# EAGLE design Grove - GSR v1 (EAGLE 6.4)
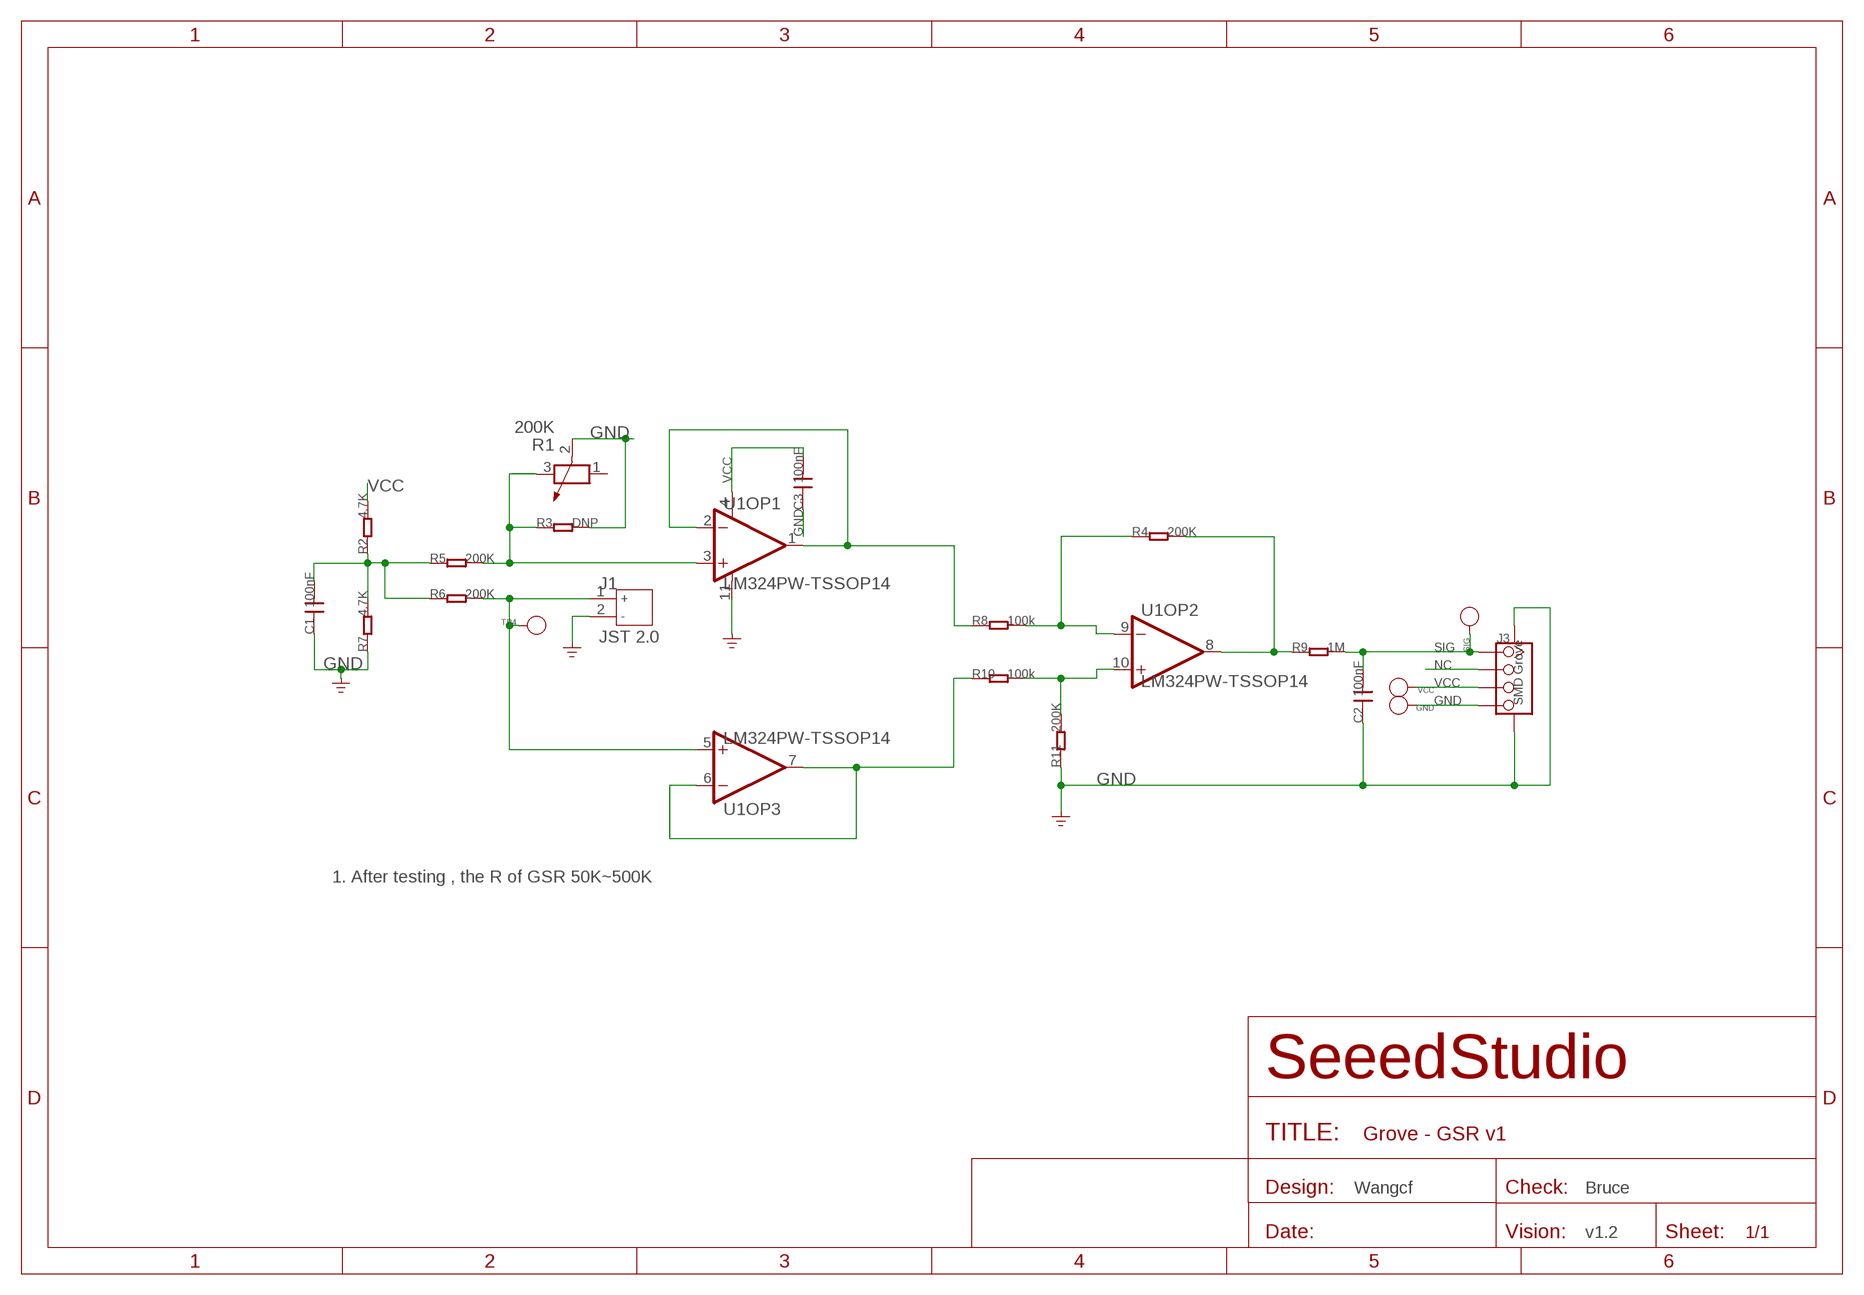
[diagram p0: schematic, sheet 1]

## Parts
C1  100nF  C-0603  [0603]
C2  100nF  C-0603  [0603]
C3  100nF  C-0603  [0603]
GND  PAD-TEST-POINT'4545'  [TP_4545]
J1  JST 2.0  JACK-JST-2P-PW'2.0'  [JST-2.0]
J3  SMD Grove  TWIG-4P-2.0-SMD-FEMALE-REINFORCE'DD'  [4P-SMD-2.0]
R1  200K  R-POTENTIOMETER-SMD  [3P-SMD-RECT-3.3X3.6]
R2  4.7K  R-0603  [0603]
R3  DNP  R-0603  [0603]
R4  200K  R-0603  [0603]
R5  200K  R-0603  [0603]
R6  200K  R-0603  [0603]
R7  4.7K  R-0603  [0603]
R8  100k  R-0603  [0603]
R9  1M  R-0603  [0603]
R10  100k  R-0603  [0603]
R11  200K  R-0603  [0603]
SIG  PAD-TEST-POINT'4545'  [TP_4545]
TP4  PAD-TEST-POINT'4545'  [TP_4545]
U1  LM324PW-TSSOP14  LMV324-TSSOP14  [TSSOP14]
VCC  PAD-TEST-POINT'4545'  [TP_4545]

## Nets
GND: C1.1 C2.1 C3.1 GND.T J1.2 J3.4 J3.SS1 J3.SS2 R1.2 R3.2 R7.1 R11.1 U1.11(OP1:V-)
IN: J1.1 R6.2 TP4.T U1.5(OP3:IN+)
N$1: R8.1 U1.1(OP1:OUT) U1.2(OP1:IN-)
N$2: R10.1 U1.6(OP3:IN-) U1.7(OP3:OUT)
N$3: R4.1 R8.2 U1.9(OP2:IN-)
N$4: R4.2 R9.1 U1.8(OP2:OUT)
N$5: R10.2 R11.2 U1.10(OP2:IN+)
N$6: C1.2 R2.1 R5.1 R6.1 R7.2
N$8: R1.3 R3.1 R5.2 U1.3(OP1:IN+)
NC: J3.2
SIG: C2.2 J3.1 R9.2 SIG.T
VCC: C3.2 J3.3 R2.2 U1.4(OP1:V+) VCC.T
Unconnected: R1.1 U1.12(OP4:IN+) U1.13(OP4:IN-) U1.14(OP4:OUT)

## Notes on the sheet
- 1. After testing , the R of GSR 50K~500K
- Wangcf | Bruce
- v1.2

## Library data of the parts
C1-C3 = Discreter:C*: Ceramic Capacitors
GND SIG TP4 VCC = Discrete:PAD-TEST-POINT; PARTNO: DNP
J1 = Connector:JACK-JST-2P-PW
J3 = Connector:TWIG-4P-2.0-SMD-FEMALE-REINFORCE
R1 = Discreter:R-POTENTIOMETER*: Potentiometer
R2-R11 = Discreter:R*
U1 = IC:LMV324: General purpose LOW Voltage, Rail-to-Rail Output Amplifiers http://www.fairchildsemi.com/ds/LM/LMV358.pdf

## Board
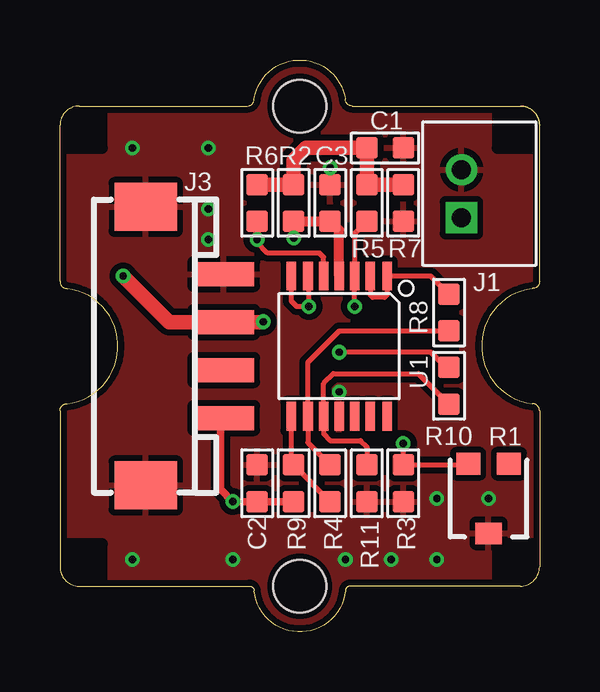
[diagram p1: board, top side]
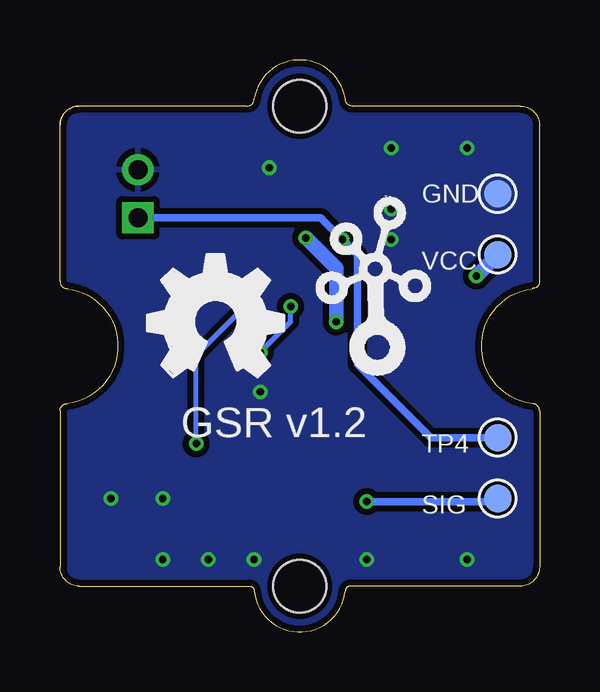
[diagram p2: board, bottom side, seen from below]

Size 20 x 23.83 mm. Coordinates in mm from the lower left corner, seen from the top.
Copper layers (1*16): Top 0.035mm / dielectric 1.5mm / Bottom 0.035mm
Design rules "SeeedStudio_rule_no_angle_090911 *": minimum track width 6mil, minimum drill 12mil, track to track 6mil, track to pad 6mil, pad to pad 6mil, via to via 6mil, smd to smd 0mil, copper to edge 10mil, drill to drill 10mil, minimum pad ring 10mil, minimum via ring 6mil, stop-mask expansion 2mil, vias tented up to drill 100mil, thermal gap 10mil

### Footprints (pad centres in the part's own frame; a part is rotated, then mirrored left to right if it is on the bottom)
0603 = smd 0.889 x 0.889: 1 -0.762,0; 2 0.762,0
TP_4545 = smd 1.143 x 1.143: T 0,0
JST-2.0 = drill 0.8 pad 1.3 square: 1 -1,0.75 | drill 0.8 pad 1.3: 2 1,0.75
4P-SMD-2.0 = smd 1 x 2.54: 1 -3,0; 2 -1,0; 3 1,0; 4 3,0 | smd 2 x 2.6: SS1 -5.8,3.25; SS2 5.8,3.25
3P-SMD-RECT-3.3X3.6 = smd 1 x 0.9: 1 -0.85,-1.45; 3 0.85,-1.45 | smd 1.1 x 0.9: 2 0,1.45
TSSOP14 = smd 0.4 x 1.2: 1 -2,-2.925; 2 -1.3,-2.925; 3 -0.65,-2.925; 4 0,-2.925; 5 0.65,-2.925; 6 1.3,-2.925; 7 2,-2.925; 8 2,2.925; 9 1.3,2.925; 10 0.65,2.925; 11 0,2.925; 12 -0.65,2.925; 13 -1.3,2.925; 14 -2,2.925
1U-DIM-W/-DRILL = hole 2.2: 0,-10; 0,10

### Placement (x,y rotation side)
C1  13.56,20.16 180 top
C2  8.22,6.19 270 top
C3  11.27,17.88 270 top
GND  1.74,18.26 0 bottom
J1  17.49,18.26 90 top
J3  6.83,11.91 90 top
R1  17.87,5.56 180 top
R2  9.75,17.88 270 top
R3  14.32,6.19 270 top
R4  11.27,6.19 270 top
R5  12.79,17.88 270 top
R6  8.22,17.88 270 top
R7  14.32,17.88 90 top
R8  16.22,13.31 270 top
R9  9.75,6.19 270 top
R10  16.22,10.26 270 top
R11  12.79,6.19 90 top
SIG  1.74,5.56 0 bottom
TP4  1.74,8.1 0 bottom
U1  11.64,11.91 180 top
U$7  [TWIGLOGO]  6.83,11.65 0 bottom
U$8  [OSHW_FILLX200_NOTEXT]  16.35,10.64 0 bottom
U$9  [1U-DIM-W/-DRILL]  10,11.91 0 top
VCC  1.74,15.72 0 bottom

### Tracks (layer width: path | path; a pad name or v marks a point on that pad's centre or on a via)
GND  (via drill 0.3 pad 0.51)
  other vias: 11.27,19.34 15.71,3.02 17.87,5.56 15.71,5.56 13.81,3.02 11.9,3.02 7.21,3.02 3.01,3.02 6.19,16.35 6.19,17.62 6.19,20.16 3.01,20.16 11.65,10
  pour Bottom (isolate 0.254): -0.16,23.97 20.29,23.97 20.29,-0.16 -0.16,-0.16
  pour Top (isolate 0.254): -0.16,23.97 20.29,23.97 20.29,-0.16 -0.16,-0.16
IN  (via drill 0.3 pad 0.51)
  Top 0.203: U1.5 10.99,15.62 10.83,15.78 8.67,15.78 8.22,16.23 v8.22,16.35 | 8.22,16.99 R6.2
  Top 0.305: v8.22,16.35 8.22,16.99
  Bottom 0.305: TP4.T 4.54,8.1 7.59,11.15 7.59,15.72 v8.22,16.35 9.05,17.18 9.1,17.23 9.13,17.26 J1.1
N$1
  Top 0.203: U1.2 12.94,14.05 13.05,13.94 13.54,13.94 13.64,14.05 U1.1 15.46,14.83 R8.1
N$2  (via drill 0.3 pad 0.51)
  Top 0.203: R10.1 16.1,11.02 15.46,11.65 v11.65,11.65 | U1.6 10.38,14.79 v10.38,13.56 9.87,13.56 9.64,13.79 U1.7
  Bottom 0.203: v11.65,11.65 10.38,12.92 v10.38,13.56
N$3
  Top 0.203: R8.2 11.65,12.54 10.34,11.23 U1.9 10.34,7.88 R4.1
N$4
  Top 0.203: U1.8 9.64,7.06 R9.1 R4.2
N$5
  Top 0.203: R10.2 14.95,10.77 11.4,10.77 10.99,10.36 U1.10 10.99,8.25 11.27,7.97 12.54,7.97 12.79,7.72 R11.2
N$6
  Top 0.61: R7.2 R5.1 C1.2 10.25,20.16 9.75,19.66 R2.1 R6.1
N$8  (via drill 0.3 pad 0.51)
  Top 0.203: R5.2 12.29,16.61 U1.3 v12.29,13.56 | R1.3 16.97,6.96 R3.1 v14.32,7.84
  Bottom 0.203: v14.32,7.84 14.32,11.53 v12.29,13.56
SIG  (via drill 0.3 pad 0.51)
  Top 0.203: 6.7,8.78 J3.1
  Top 0.305: 6.7,8.78 6.7,5.94 v7.21,5.43 C2.2 R9.2
  Bottom 0.305: v7.21,5.43 2.13,5.43 1.87,5.69 SIG.T
VCC  (via drill 0.3 pad 0.51)
  Top 0.406: U1.4 11.64,16.74 C3.2 R2.2 v9.75,16.42
  Top 0.61: v8.48,12.92 8.46,12.91 J3.3 4.55,12.91 v2.63,14.83
  Bottom 0.61: v8.48,12.92 8.48,15.15 v9.75,16.42 | v2.63,14.83 VCC.T

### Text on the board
bPlace: GSR v1.2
